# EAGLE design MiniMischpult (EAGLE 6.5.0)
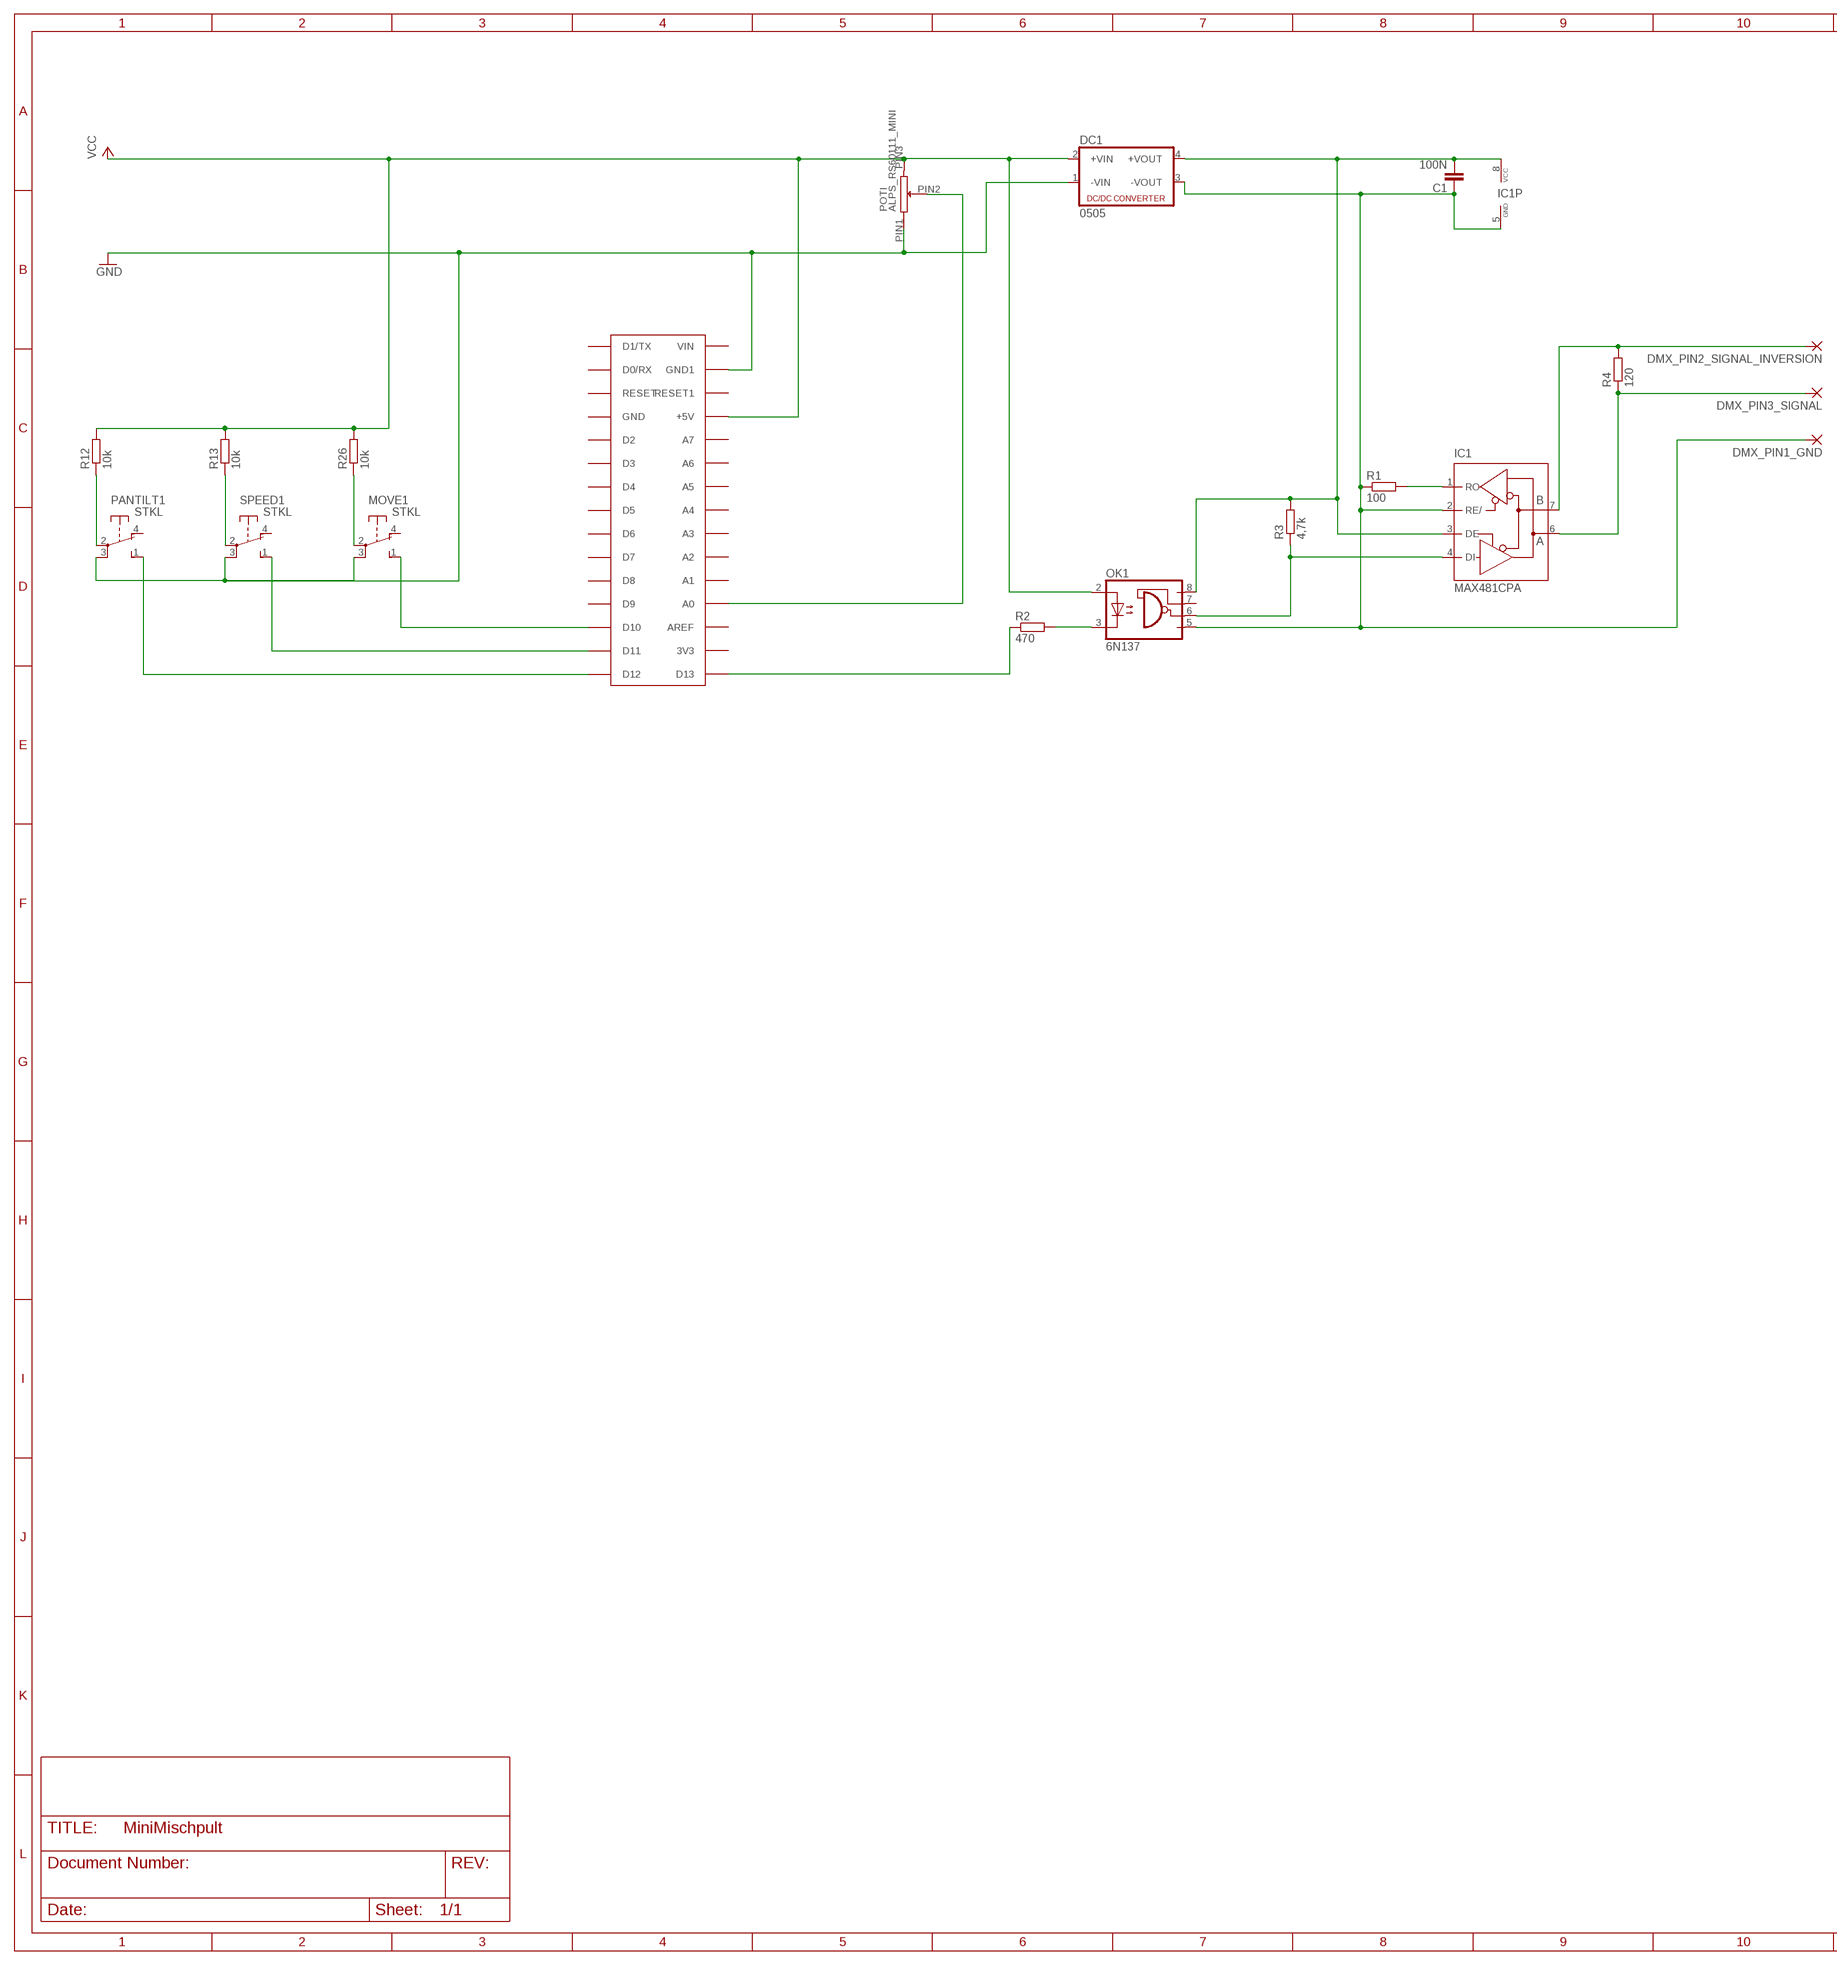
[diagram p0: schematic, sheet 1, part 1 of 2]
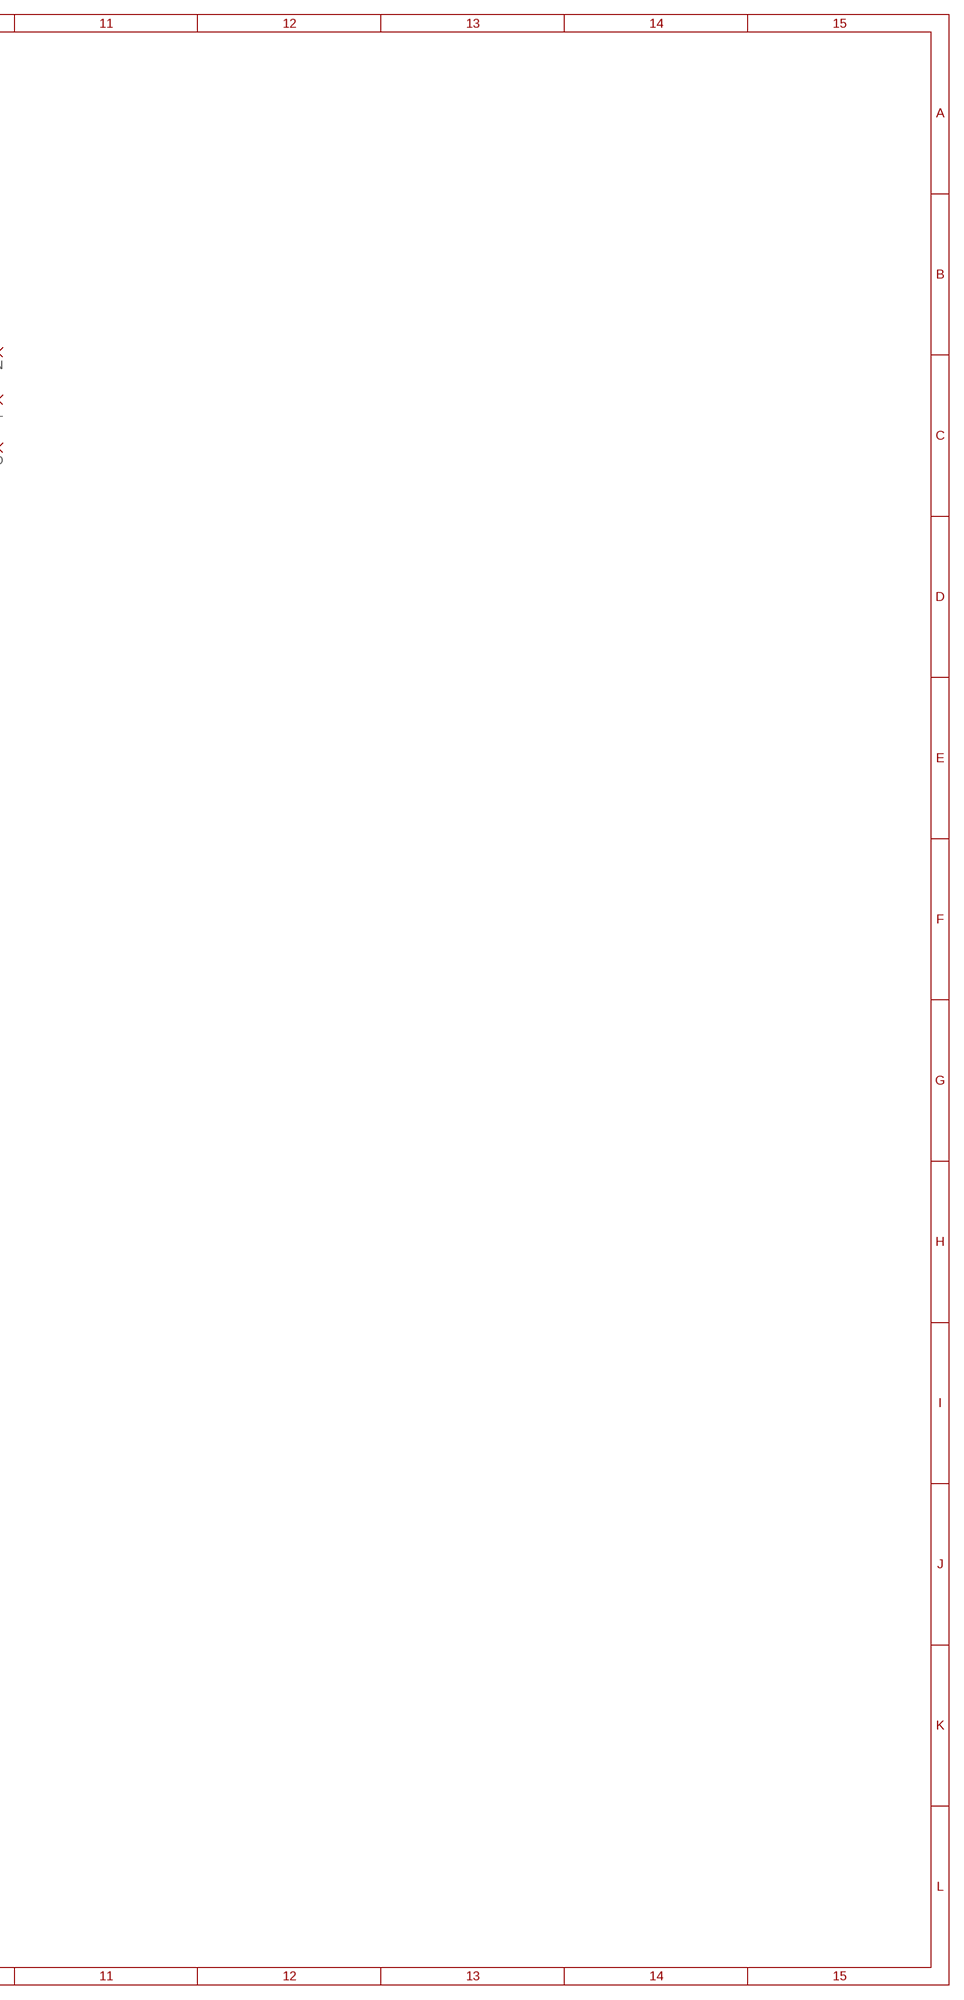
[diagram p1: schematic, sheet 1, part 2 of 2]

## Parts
C1  100N  C-EUC1206  [C1206]
DC1  0505  NME  [NME]
DMX_PIN1_GND  2,54/1,1  [2,54/1,1]
DMX_PIN2_SIGNAL_INVERSION  2,54/1,1  [2,54/1,1]
DMX_PIN3_SIGNAL  2,54/1,1  [2,54/1,1]
IC1  MAX481CPA  [DIL08]
MOVE  STKL  [STKL]
OK1  6N137  [DIL08]
PANTILT  STKL  [STKL]
POTI  ALPS_RS60111_MINI  [ALPS_RS60112_60MM_STEREO_MINI]
R1  100  R-EU_M1206  [M1206]
R2  470  R-EU_M1206  [M1206]
R3  4,7k  R-EU_M1206  [M1206]
R4  120  R-EU_M1206  [M1206]
R12  10k  R-EU_R1206  [R1206]
R13  10k  R-EU_R1206  [R1206]
R26  10k  R-EU_R1206  [R1206]
SPEED  STKL  [STKL]
U$1  ARDUINONANO1,1MM-BOHRUNG  [PDIP-32GROSSE-BOHRUNG]

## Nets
GND: DC1.1(-VIN) MOVE.3(1:P) PANTILT.3(1:P) POTI.PIN1 SPEED.3(1:P) U$1.GND1
GND2: C1.1 DC1.3(-VOUT) DMX_PIN1_GND.1(P) IC1.2(RE/) IC1.5(GND) OK1.5(GND) R1.1
N$1: R2.1 U$1.D13
N$2: PANTILT.2(1:P) R12.1
N$3: POTI.PIN2 U$1.A0
N$6: R13.1 SPEED.2(1:P)
N$7: MOVE.2(1:P) R26.1
N$9: PANTILT.1(1:S) U$1.D12
N$10: SPEED.1(1:S) U$1.D11
N$11: MOVE.1(1:S) U$1.D10
N$32: IC1.1(RO) R1.2
N$34: IC1.4(DI) OK1.6(VO) R3.1
N$36: DMX_PIN3_SIGNAL.1(P) IC1.6(A) R4.1
N$37: DMX_PIN2_SIGNAL_INVERSION.1(P) IC1.7(B) R4.2
N$41: OK1.3(C) R2.2
VCC: DC1.2(+VIN) OK1.2(A) POTI.PIN3 R12.2 R13.2 R26.2 U$1.+5V
VCC2: C1.2 DC1.4(+VOUT) IC1.3(DE) IC1.8(VCC) OK1.8(VCC) R3.2
Unconnected: MOVE.4(1:O) MOVE.+(D1:A) MOVE.-(D1:C) OK1.7(VE) PANTILT.4(1:O) PANTILT.+(D1:A) PANTILT.-(D1:C) SPEED.4(1:O) SPEED.+(D1:A) SPEED.-(D1:C) U$1.3V3 U$1.A1 U$1.A2 U$1.A3 U$1.A4 U$1.A5 U$1.A6 U$1.A7 U$1.AREF U$1.D0/RX U$1.D1/TX U$1.D2 U$1.D3 U$1.D4 U$1.D5 U$1.D6 U$1.D7 U$1.D8 U$1.D9 U$1.GND U$1.RESET U$1.RESET1 U$1.VIN

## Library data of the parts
C1 = rcl:C-EU: CAPACITOR, European symbol
DC1 = dc-dc-converter:NME: DC-DC CONVERTER; MF: C & D TECHNOLOGIES, INC; MPN: NME1205D; OC_FARNELL: 1021466; OC_NEWARK: 98B8198
DMX_PIN1_GND DMX_PIN2_SIGNAL_INVERSION DMX_PIN3_SIGNAL = wirepad:2,54/1,1: THROUGH-HOLE PAD
IC1 = maxim:MAX481CPA: RS485 TRANSEIVER; MPN: MAX481CPA+; OC_FARNELL: unknown; OC_NEWARK: 99K3445
MOVE PANTILT SPEED = switch-misc:STKL: SWITCH
OK1 = optocoupler:6N137: MOTOROLA OPTO COUPLER; MPN: 6N137; OC_FARNELL: 1328376; OC_NEWARK: 52M1895
POTI = ALPS-SchiebePoti:ALPS_RS60111_MINI: ALPS RS60112 60MM MONO Der MONO-Fader hat alle Anschluesse die auch der Stereo hat, verwendet jedoch 3 davon nicht. Es wird also nur ein Kanal verwendet. Auch die Fader ohne Befestigungen (die beiden mittleren Bohrloecher) sind kompatibel mit dieser Bibliothek
R1-R4 R12 R13 R26 = rcl:R-EU_: RESISTOR, European symbol
U$1 = arduino:ARDUINONANO

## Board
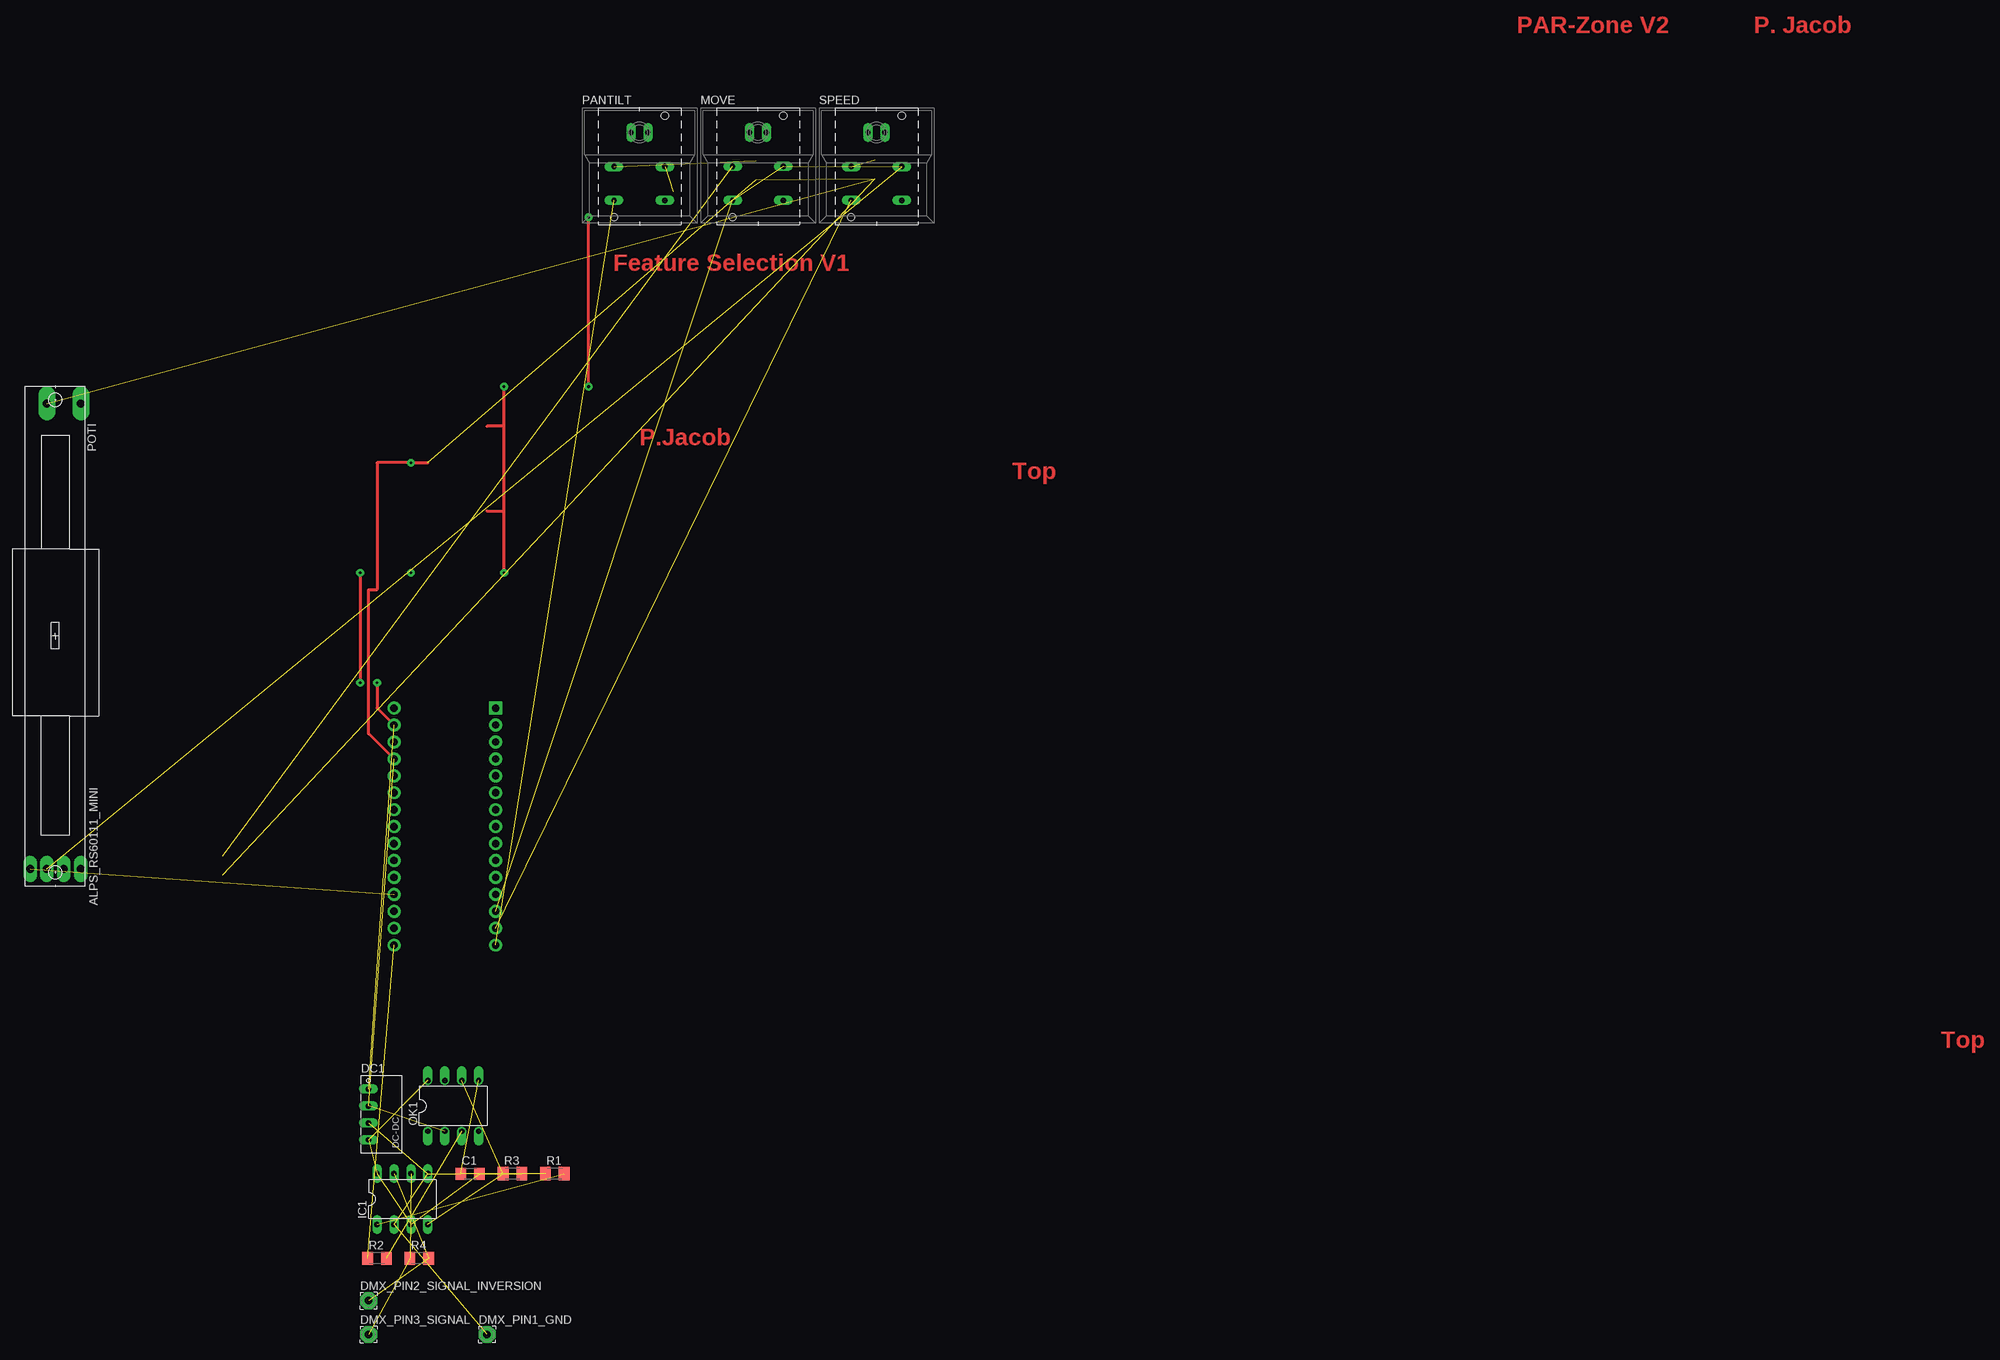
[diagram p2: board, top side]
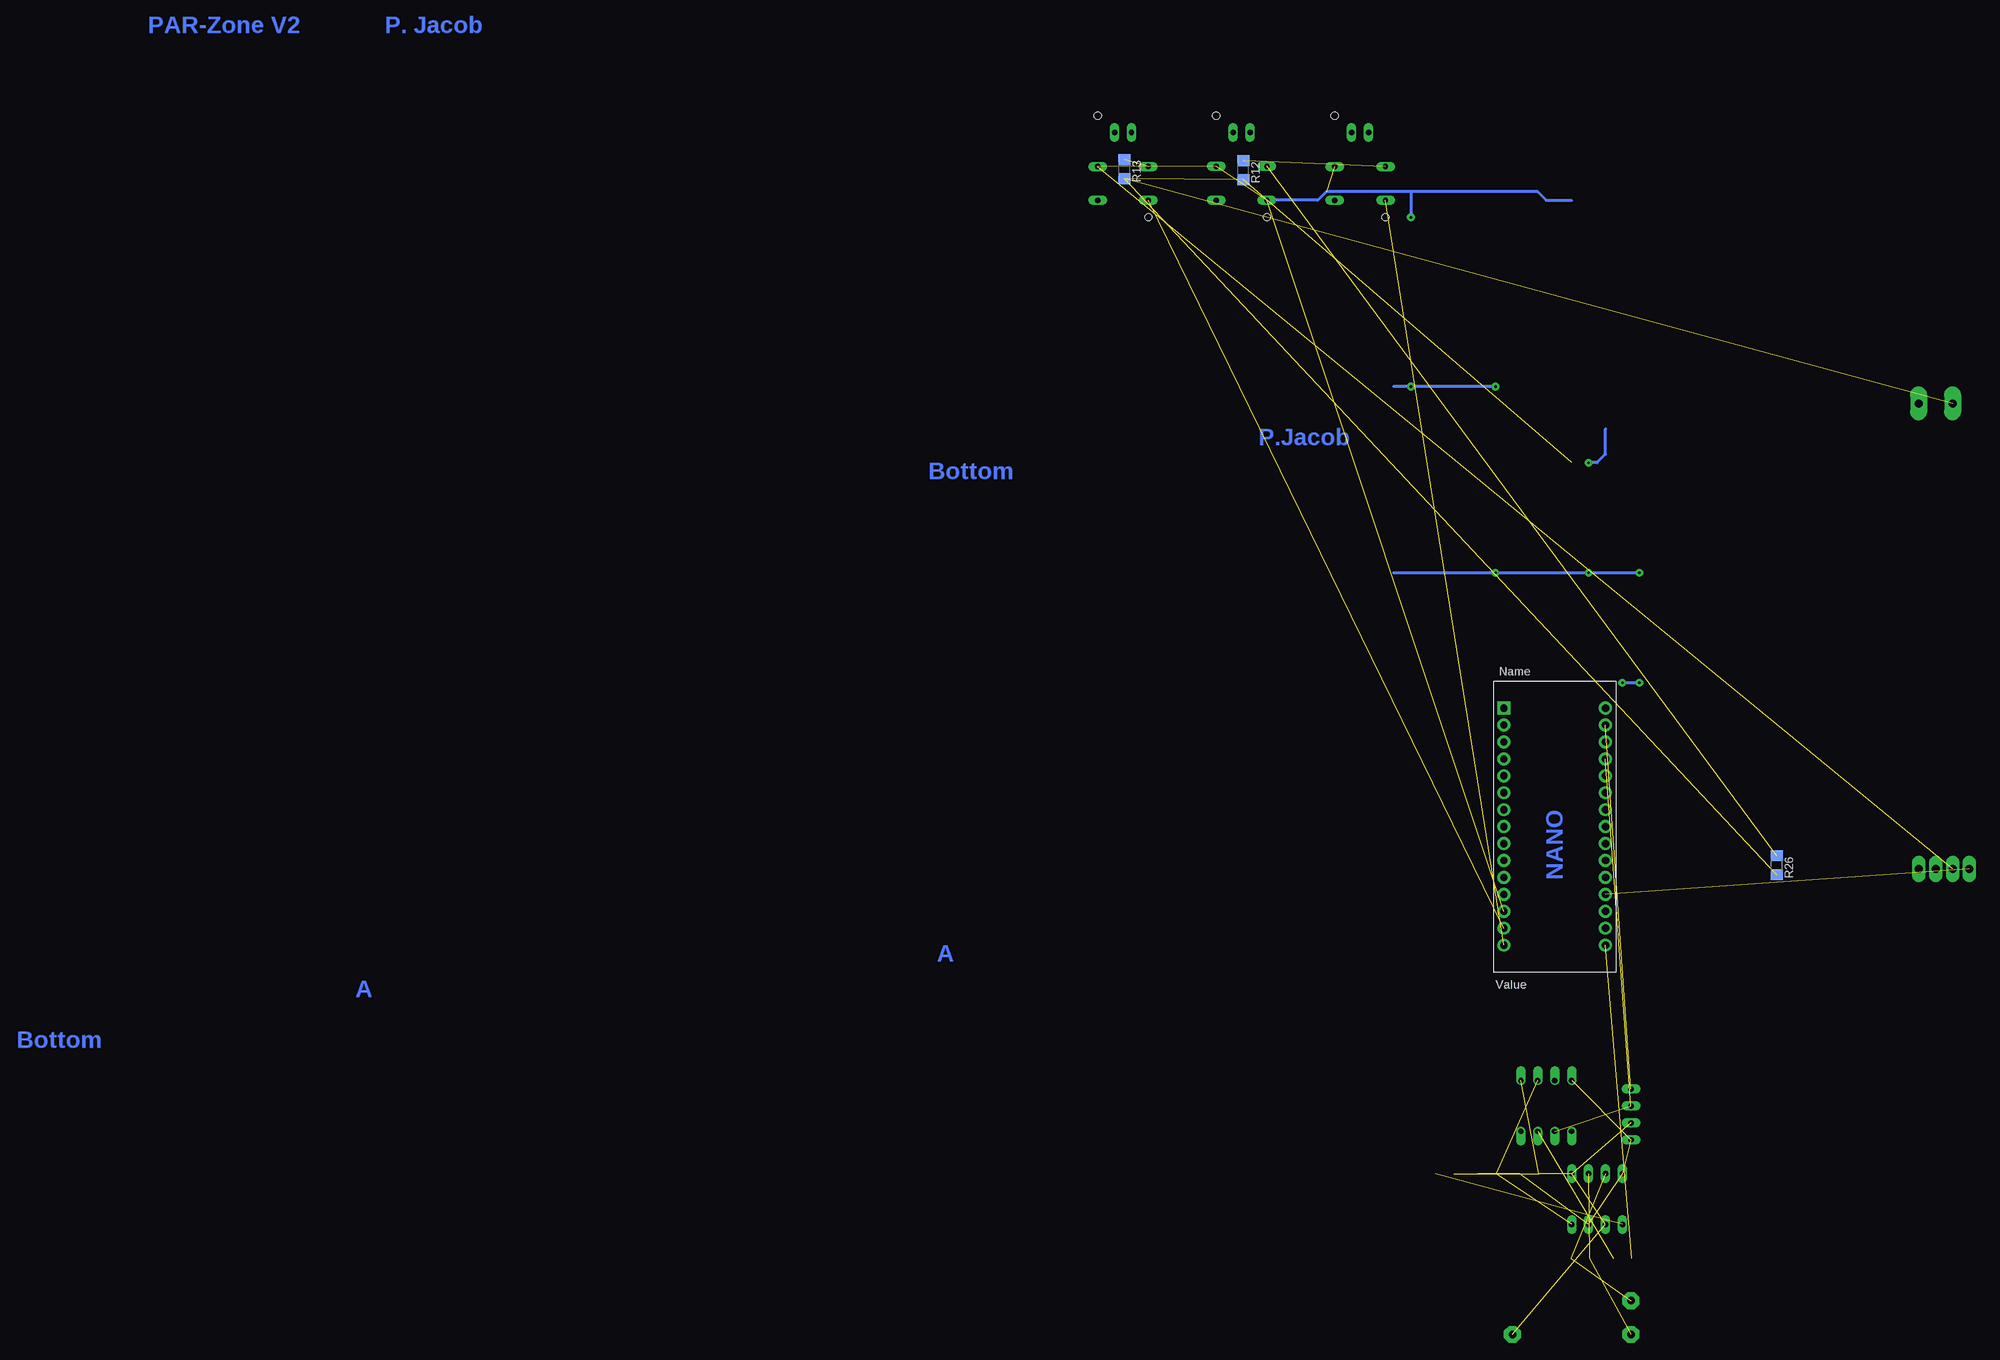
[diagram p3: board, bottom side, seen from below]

No outline drawn. Coordinates in mm, seen from the top.
Copper layers (1*16): Top 0.035mm / dielectric 1.5mm / Bottom 0.035mm
Design rules "HTWG Sinnvoll": minimum track width 18mil, minimum drill 0.4mm, track to track 12mil, track to pad 12mil, pad to pad 18mil, via to via 18mil, smd to smd 18mil, copper to edge 40mil, drill to drill 8mil, minimum pad ring 12mil, minimum via ring 15mil, stop-mask expansion 4mil, vias tented up to drill 0mil, thermal gap 10mil

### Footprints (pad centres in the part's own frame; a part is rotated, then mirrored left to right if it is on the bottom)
C1206 = smd 1.6 x 1.8: 1 -1.4,0; 2 1.4,0
NME = drill 0.813 long: 1 0,3.81; 2 0,1.27; 3 0,-1.27; 4 0,-3.81
2,54/1,1 = drill 1.118 pad 2.54 octagon: 1 0,0
DIL08 = drill 0.813 long: 1 -3.81,-3.81; 2 -1.27,-3.81; 3 1.27,-3.81; 4 3.81,-3.81; 5 3.81,3.81; 6 1.27,3.81; 7 -1.27,3.81; 8 -3.81,3.81
STKL = drill 0.813 long: 1 -3.81,-5.08; 2 -3.81,0; 3 3.81,0; 4 3.81,-5.08; + -1.27,5.08; - 1.27,5.08 | hole 1.118: 3.81,7.62; -3.81,-7.62
DIL08' = drill 0.813 offset: 1 -3.81,-3.81; 2 -1.27,-3.81; 3 1.27,-3.81; 4 3.81,-3.81; 5 3.81,3.81; 6 1.27,3.81; 7 -1.27,3.81; 8 -3.81,3.81
ALPS_RS60112_60MM_STEREO_MINI = drill 1.2 pad 2 long: PIN1 5.715,72.39; PIN1' 3.175,72.39; PIN2 8.255,72.39; PIN2' 0.635,72.39 | drill 1.2 pad 2.54 long: PIN3 5.715,2.54; PIN3' 0.635,2.54
M1206 = smd 1.6 x 2: 1 -1.4,0; 2 1.4,0
R1206 = smd 1.6 x 1.803: 1 -1.422,0; 2 1.422,0
PDIP-32GROSSE-BOHRUNG = drill 1.1 pad 1.93: 3V3 15.24,-35.56; +5V 15.24,-10.16; A0 15.24,-30.48; A1 15.24,-27.94; A2 15.24,-25.4; A3 15.24,-22.86; A4 15.24,-20.32; A5 15.24,-17.78; A6 15.24,-15.24; A7 15.24,-12.7; AREF 15.24,-33.02; D0/RX 0,-5.08; D2 0,-12.7; D3 0,-15.24; D4 0,-17.78; D5 0,-20.32; D6 0,-22.86; D7 0,-25.4; D8 0,-27.94; D9 0,-30.48; D10 0,-33.02; D11 0,-35.56; D12 0,-38.1; D13 15.24,-38.1; GND 0,-10.16; GND1 15.24,-5.08; RESET 0,-7.62; RESET1 15.24,-7.62; VIN 15.24,-2.54 | drill 1.1 pad 1.93 square: D1/TX 0,-2.54

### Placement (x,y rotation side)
C1  22.86,-16.51 0 top
DC1  7.62,-7.62 0 top
DMX_PIN1_GND  25.4,-40.64 0 top
DMX_PIN2_SIGNAL_INVERSION  7.62,-35.56 0 top
DMX_PIN3_SIGNAL  7.62,-40.64 0 top
IC1  12.7,-20.32 0 top
MOVE  66.04,134.63 0 top
OK1  6N137  [DIL08']  20.32,-6.35 0 top
PANTILT  48.26,134.62 0 top
POTI  -34.92,101.6 180 top
R1  35.56,-16.51 0 top
R2  8.89,-29.21 0 top
R3  29.21,-16.51 0 top
R4  15.24,-29.21 0 top
R12  65.79,134.06 270 bottom
R13  83.61,134.21 270 bottom
R26  -14.25,29.76 270 bottom
SPEED  83.82,134.62 0 top
U$1  26.67,55.88 0 bottom

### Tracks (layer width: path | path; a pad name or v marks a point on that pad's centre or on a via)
GND  (via drill 0.4)  (5 unrouted)
  Top 0.457: 27.94,95.63 25.4,95.63 | 27.94,82.93 27.94,95.63 | 25.4,82.93 27.94,82.93 | v8.89,57.15 8.89,53.34 U$1.GND1 | v6.35,73.66 v6.35,57.15 | v27.94,73.66 27.94,82.93 | 27.94,95.63 v27.94,101.6 | v40.64,101.6 v40.64,127
  Bottom 0.457: 16.51,129.54 20.32,129.54 21.59,130.81 40.64,130.81 | 40.64,130.81 v40.64,127 | 62.23,129.54 54.61,129.54 53.34,130.81 40.64,130.81 | 43.18,73.66 v27.94,73.66 v13.97,73.66 v6.35,73.66 | v6.35,57.15 v8.89,57.15 | v27.94,101.6 v40.64,101.6 43.18,101.6
GND2  (6 unrouted)
N$1  (1 unrouted)
N$2  (1 unrouted)
N$3  (1 unrouted)
N$6  (1 unrouted)
N$7  (1 unrouted)
N$9  (1 unrouted)
N$10  (1 unrouted)
N$11  (1 unrouted)
N$32  (1 unrouted)
N$34  (2 unrouted)
N$36  (2 unrouted)
N$37  (2 unrouted)
N$41  (1 unrouted)
VCC  (via drill 0.4)  (6 unrouted)
  Top 0.457: U$1.+5V 7.62,49.53 7.62,71.12 8.89,71.12 8.89,90.17 v13.97,90.17 16.51,90.17
  Bottom 0.457: 11.43,95.25 11.43,91.44 12.7,90.17 v13.97,90.17
VCC2  (5 unrouted)

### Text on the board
Top: PAR-Zone V2 P. Jacob | Feature Selection V1 | P.Jacob | Top | Top
Bottom: PAR-Zone V2 P. Jacob | P.Jacob | Bottom | NANO | A | A | Bottom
